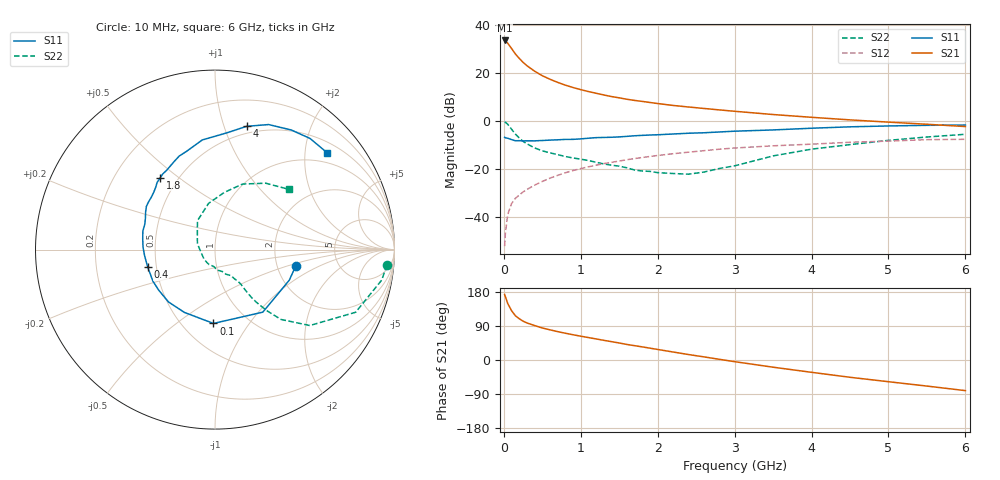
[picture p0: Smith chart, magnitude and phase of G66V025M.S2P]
! SIEMENS Small Signal Semiconductors
! BFG193
! Si NPN RF Bipolar Junction Transistor in SOT223
! VCE = 6 V  IC = 25 mA
! Common Emitter S-Parameters:  August  1996
# GHz  S  MA  R  50
!  f  S11  S21  S12  S22
! GHz  MAG  ANG  MAG  ANG  MAG  ANG  MAG  ANG
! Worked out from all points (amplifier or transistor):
!   36 points, 10 MHz to 6 GHz, reference 50 ohm
!   highest |S21| = 33.5 dB at 10 MHz (marker M1)
!   |S21| within 3 dB of that: start of sweep to 92.45 MHz
!   unconditionally stable (mu >= 1): 657 MHz to 2.512 GHz
!   at 250 MHz: K = 0.79, MSG = 27.0 dB, |S12| = -29.5 dB
!   at 1.4 GHz: K = 1.05, MAG = 12.3 dB, |S12| = -17.2 dB
!   at 6 GHz: K = 0.88, MSG = 2.7 dB, |S12| = -7.6 dB
!   S11 on the Smith chart (normalised r, x): 10 MHz: 2.54, -0.58; 100 MHz: 0.70, -0.69; 400 MHz: 0.45, -0.10; 1.8 GHz: 0.40, +0.43; 4 GHz: 0.43, +1.19; 6 GHz: 0.74, +2.50
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0.01  0.4593 -11.3  47.39 172.8  0.0025 88.7  0.9618 -5.1
0.02  0.4476 -22.4  46.24 167.2  0.0046 81.8  0.944 -10.4
0.05  0.4387 -52.6  41.6 149.4  0.0113 73.2  0.8579 -24.0
0.1  0.4115 -91.2  32.29 130.3  0.0192 65.0  0.6767 -38.7
0.15  0.3893 -116.0  24.85 116.8  0.0247 61.0  0.5357 -46.6
0.2  0.3902 -131.6  20.1 108.9  0.0289 60.9  0.4464 -49.7
0.25  0.3866 -143.9  16.62 102.5  0.0335 61.5  0.3778 -51.7
0.3  0.3881 -152.9  14.16 97.8  0.0378 62.7  0.3362 -52.7
0.4  0.3874 -165.2  10.87 90.9  0.0464 63.1  0.2759 -53.2
0.5  0.394 -175.3  8.764 84.5  0.0555 62.9  0.2402 -53.2
0.6  0.4014 178.0  7.392 79.6  0.0649 63.0  0.218 -54.1
0.7  0.407 171.6  6.363 74.9  0.0743 62.1  0.2002 -55.9
0.9  0.4159 160.2  4.975 66.6  0.0935 59.7  0.1706 -58.3
1.1  0.4394 151.6  4.102 59.2  0.1116 56.8  0.1508 -65.7
1.4  0.4602 140.1  3.228 48.4  0.1384 51.3  0.1207 -77.4
1.8  0.5036 127.2  2.56 34.6  0.1746 43.5  0.0915 -100.0
2.2  0.5375 115.7  2.11 21.1  0.2094 34.6  0.0811 -138.4
3.5  0.6529 84.4  1.366 -19.0  0.3053 4.4  0.1883 121.3
4  0.7091 75.6  1.196 -32.5  0.3306 -5.3  0.2601 97.9
4.5  0.758 66.8  1.057 -45.6  0.3618 -15.4  0.3233 80.7
5.5  0.8146 49.5  0.857 -68.8  0.4101 -38.8  0.4656 52.6
6  0.8256 40.8  0.768 -80.8  0.4171 -52.3  0.5305 39.3
